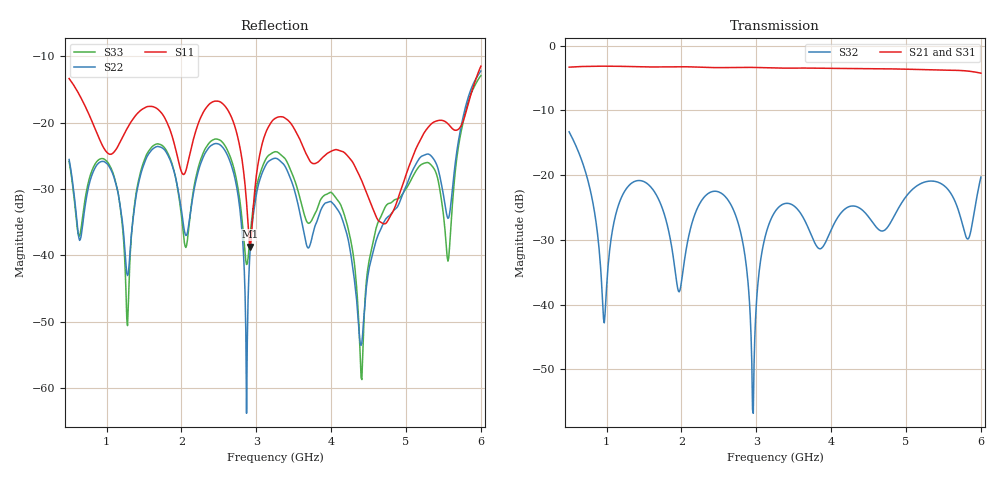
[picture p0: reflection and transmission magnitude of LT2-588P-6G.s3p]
! MTS Systemtechnik GmbH
! S-Parameters
! Model: LT2-588P-6G
! Rohde & Schwarz ZVB8 2Ports - Version 3.20 - 1145.1010k08 SN: 100119
! Converted & adapted with MATLAB
!		|  MTS  |
!		|  |--o OUT 2 (Port 3)
! C (Port 1) o--| LT2-588P-6G |
!		|  |--o OUT 1 (Port 2)
! S3P File: Measurements:
! <S11,S12,S13>,
! <S21,S22,S23>,
! <S31,S32,S33>:
# HZ  S  DB  R  50.00
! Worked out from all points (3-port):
!   551 points, 500 MHz to 6 GHz, reference 50 ohm
!   strongest paths, dB at 500 MHz, 1.87 GHz, 3.25 GHz, 4.63 GHz, 6 GHz:
!     S21: -3.3, -3.3, -3.4, -3.6, -4.2
!     S31: -3.3, -3.3, -3.4, -3.6, -4.3
!     S32: -13.3, -31.1, -25.6, -28.4, -20.3
!   lowest |S11| = -38.7 dB at 2.92 GHz (marker M1), VSWR 1.02, Z = 48.9 - j0.245 ohm
!   |S11| at or under -10 dB: start of sweep to end of sweep
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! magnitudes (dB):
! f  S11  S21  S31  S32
! 500 MHz  -13.4  -3.3  -3.3  -13.3
! 970 MHz  -24.0  -3.2  -3.2  -42.8
! 1.28 GHz  -20.8  -3.2  -3.2  -21.8
! 1.44 GHz  -18.3  -3.2  -3.2  -20.8
! 2.58 GHz  -17.5  -3.4  -3.4  -23.2
! 2.92 GHz  -38.7  -3.3  -3.3  -41.9
! 3.25 GHz  -19.4  -3.4  -3.4  -25.6
! 4.14 GHz  -24.3  -3.5  -3.5  -25.7
! 4.4 GHz  -28.5  -3.5  -3.6  -25.2
! 6 GHz  -11.5  -4.2  -4.3  -20.3
